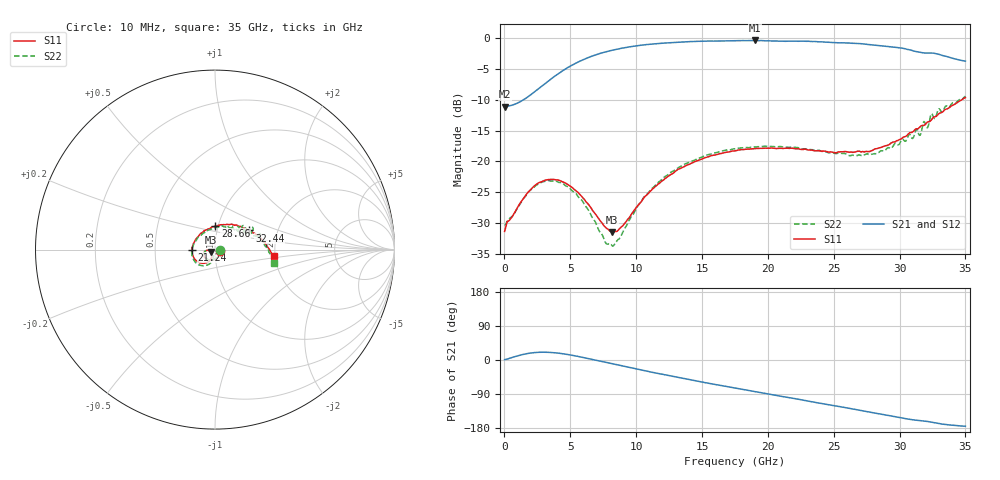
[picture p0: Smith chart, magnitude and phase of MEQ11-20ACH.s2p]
! MARKI MICROWAVE INC.
! Email:  support@markimicrowave.com  Phone:  408-778-4200
! Model Number:  MEQ11-20ACH  Date:  6/18
! Filename:		MEQ11-20ACH.S2P  Version: 1.0
! Description:  2-port S-parameter data for chip equalizer
! Features:		Low Insertion Loss, Excellent Return Loss
! Frequency Measured: 	10 MHz to 35 GHz
! S2P File: Measurements: S11, S21, S12, S22:
# Hz S  dB  R 50
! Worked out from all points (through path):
!   1601 points, 10 MHz to 35 GHz, reference 50 ohm
!   highest |S21| = -0.39 dB at 19.04 GHz (marker M1); lowest = -11.1 dB at 10 MHz (marker M2)
!   lowest |S11| = -31.4 dB at 8.167 GHz (marker M3), VSWR 1.06, Z = 47.7 - j1.3 ohm
!   |S11| at or under -10 dB: start of sweep to 34.73 GHz
!   |S22| runs from -33.7 to -9.4 dB; largest |S21 - S12| = 0.01
!   S11 on the Smith chart (normalised r, x): 10 MHz: 1.05, -0.01; 21.24 GHz: 0.77, -0.00; 28.66 GHz: 0.97, +0.26; 32.44 GHz: 1.43, +0.32; 35 GHz: 1.96, -0.17
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1e7  -31.34 -12.4  -11.13 1.1  -10.97 1.6  -30.38 -4.9
1.628288e9  -25.43 -90.1  -9.75 16.3  -9.75 16.3  -25.56 -90.2
2.743594e9  -23.32 -123.3  -7.94 20.4  -7.94 20.5  -23.45 -123.2
4.340012e9  -23.22 -155.6  -5.40 16.9  -5.41 16.9  -23.43 -156.4
5.848956e9  -25.61 -172.7  -3.62 7.6  -3.62 7.6  -26.21 -175.1
7.685931e9  -30.70 -162.2  -2.24 -6.0  -2.23 -6.1  -33.16 -159.4
8.167044e9  -31.40 -149.6  -1.98 -9.7  -1.98 -9.7  -33.66 -138.4
8.954319e9  -30.47 -128.3  -1.63 -15.7  -1.62 -15.8  -31.60 -113.1
1.0507e10  -26.14 -112.8  -1.13 -27.3  -1.12 -27.2  -26.01 -101.0
1.168791e10  -23.62 -115.4  -0.89 -35.8  -0.88 -35.7  -23.37 -104.3
1.488075e10  -19.70 -132.4  -0.51 -57.4  -0.52 -57.3  -19.38 -123.6
1.7505e10  -18.26 -150.4  -0.44 -74.0  -0.44 -74.2  -17.94 -141.4
1.903581e10  -17.91 -161.9  -0.39 -83.7  -0.40 -83.6  -17.66 -151.9
2.124456e10  -17.85 -180.0  -0.52 -97.3  -0.49 -97.6  -17.65 -168.9
2.334396e10  -18.16 161.6  -0.56 -110.2  -0.56 -110.0  -18.09 171.7
2.62525e10  -18.48 126.1  -0.82 -128.1  -0.88 -128.4  -19.07 135.6
2.865806e10  -17.65 89.0  -1.26 -143.3  -1.21 -143.6  -18.29 93.3
2.918291e10  -17.30 81.1  -1.37 -146.5  -1.35 -147.0  -17.76 83.8
3.154474e10  -14.41 43.1  -2.29 -160.0  -2.35 -159.9  -15.77 40.2
3.244136e10  -13.19 29.2  -2.44 -163.9  -2.40 -163.8  -12.25 30.1
3.357853e10  -11.50 12.4  -3.00 -170.7  -3.04 -170.9  -11.00 9.5
3.5e10  -9.65 -6.6  -3.74 -174.8  -3.79 -174.2  -9.42 -12.6
